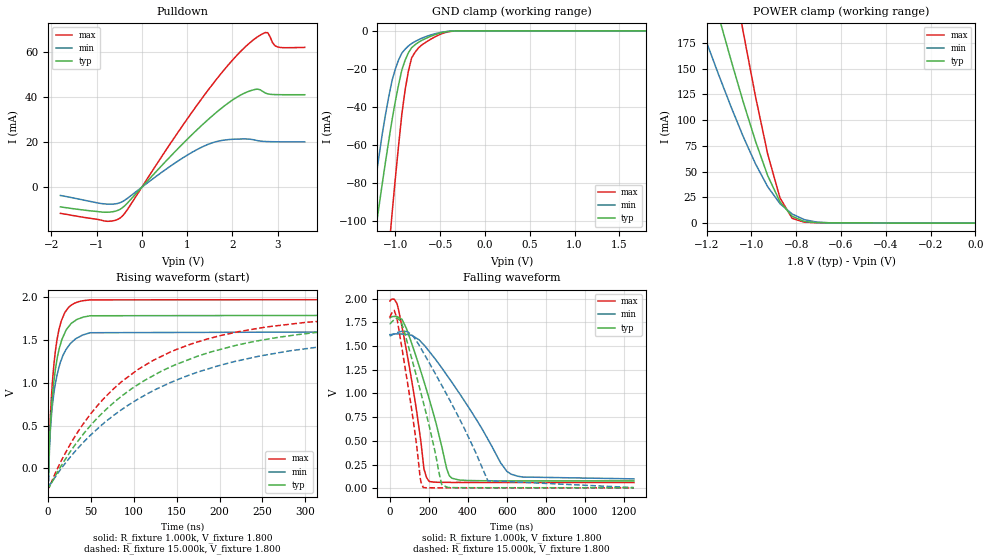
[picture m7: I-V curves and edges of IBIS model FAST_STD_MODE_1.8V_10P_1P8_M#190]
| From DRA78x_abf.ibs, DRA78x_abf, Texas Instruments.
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| Model based on original model for BI2C1833DVFZP18_SSCEV
|   Sub model FAST_STD_MODE_1.8V_10P_1P8
[model]   FAST_STD_MODE_1.8V_10P_1P8_M#190
|[Description]  [1.8V-I/O_OPEN_DRAIN-X-FAST MODE AND STD MODE, IND, 10 PERCENT%]
|   FAST MODE AND STD MODE, ,IND,10 PERCENT%
|[Input Load]
|[Output Drive] FAST MODE AND STD MODE
|Voltage   1.8V
|Mode   I/O_OPEN_DRAIN
Model_type   I/O_open_drain
Polarity   Non-Inverting
Enable   Active-Low
Vinl =  0.54
Vinh =  1.26
Cref =  15pF
Rref =  1000
Vref =  1.8V
Vmeas =  0.9
C_comp   2.29p   1.81p   2.77p
[Model Spec]
Vinl   0.54   0.486   0.594
Vinh   1.26   1.134   1.386
[Temperature Range]   25   125   -40
[Voltage Range]   1.8   1.62   1.98
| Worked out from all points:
|   slope of the pulldown table from 0 to 0.27 V, typ, clamps not added: 45.4 ohm
|   GND clamp passes 1 mA (typ) near -0.49 V on its own axis
|   POWER clamp passes 1 mA (typ) near -0.74 V on its own axis
|   rising waveform, R_fixture 1.000k, V_fixture 1.800: 20-80 % time 12.4ns typ, 14.8ns min, 10.2ns max; typ from 0.077 V to 1.8 V
|   rising waveform, R_fixture 15.000k, V_fixture 1.800: 20-80 % time 164ns typ, 193ns min, 135ns max; typ from 0.005 V to 1.73 V
|   falling waveform, R_fixture 1.000k, V_fixture 1.800: 20-80 % time 144ns typ, 283ns min, 88.9ns max; typ from 1.8 V to 0.077 V
|   falling waveform, R_fixture 15.000k, V_fixture 1.800: 20-80 % time 125ns typ, 239ns min, 77.8ns max; typ from 1.73 V to 0.005 V
[POWER_clamp]
-1.8V     746.5mA    555.3mA    1.181A
-1.218V   258.3mA    186.3mA    411.3mA
-1.127V   186.2mA    133.2mA    296.1mA
-1.055V   130.9mA    93.44mA    207.1mA
-1.036V   117.4mA    83.77mA    185.1mA
-981.8mV  79.41mA    57.45mA    122.8mA
-927.3mV  45.94mA    35.22mA    66.84mA
-872.7mV  20.67mA    18.89mA    24.46mA
-818.2mV  6.579mA    8.765mA    4.591mA
-763.6mV  1.447mA    3.292mA    765.1uA
-654.5mV  205.7uA    269.1uA    284.5uA
0V        2.27uA     701.3nA    6.122uA
[Pulldown]
-1.8V     -8.76mA    -3.66mA    -11.64mA
-763.6mV  -11.13mA   -7.517mA   -15.17mA
-490.9mV  -9.952mA   -6.962mA   -13.87mA
1.255V    26.22mA    17.12mA    37.49mA
1.691V    34.03mA    20.51mA    49.08mA
2.291V    42.09mA    21.48mA    62.55mA
2.564V    43.64mA    20.71mA    67.02mA
2.727V    41.93mA    20.35mA    68.83mA
2.782V    41.54mA    20.3mA     68.79mA
2.891V    41.26mA    20.25mA    64.24mA
3V        41.2mA     20.22mA    62.42mA
3.6V      41.16mA    20.17mA    62.23mA
[GND_clamp]
-1.8V     -312.7mA   -306.1mA   -547.2mA
-1.291V   -129.4mA   -103.7mA   -240.2mA
-1.218V   -104.5mA   -78.02mA   -197.8mA
-1.182V   -92.38mA   -65.92mA   -176.8mA
-1.073V   -57.71mA   -34.59mA   -115.9mA
-1.036V   -46.88mA   -26.15mA   -96.3mA
-927.3mV  -20.64mA   -11.73mA   -43.97mA
-890.9mV  -15.5mA    -9.682mA   -31.24mA
-818.2mV  -8.896mA   -6.689mA   -14.3mA
-672.7mV  -4.275mA   -3.291mA   -6.44mA
-381.8mV  -173.6uA   -151uA     -298.3uA
1.8V      2.27uA     911.4nA    5.692uA
[Ramp]
dV/dt_f   0.559368/0.17762757u   0.406134/0.41534074u   0.719898/0.10455527u
dV/dt_r   76.3794m/79.261671p 55.808172m/0.11582494n 92.758032m/57.986588p
R_load = 50
[Rising Waveform]
R_fixture = 1.000k
V_fixture = 1.800
V_fixture_min = 1.620
V_fixture_max = 1.980
0s        76.67mV    97.9mV     60.38mV
126ps     76.67mV    97.9mV     -142.9mV
334.9ps   -99.36mV   97.9mV     -35.5mV
768ps     77.25mV    -41.8mV    132.6mV
2.082ns   408.4mV    351.8mV    499.5mV
5.121ns   857.1mV    751mV      1.027V
12.66ns   1.385V     1.183V     1.623V
23.81ns   1.652V     1.428V     1.878V
40.96ns   1.764V     1.558V     1.956V
1.25us    1.798V     1.619V     1.974V
[Rising Waveform]
R_fixture = 15.000k
V_fixture = 1.800
V_fixture_min = 1.620
V_fixture_max = 1.980
350fs     5.398mV    6.72mV     4.165mV
147.2ps   5.398mV    6.72mV     -221.7mV
367.2ps   -210mV     6.72mV     -222.6mV
1.142ns   -213.1mV   -193.1mV   -222.1mV
45.92ns   460.5mV    353.5mV    588.3mV
104.9ns   979mV      809.5mV    1.155V
171.8ns   1.3V       1.114V     1.467V
254.1ns   1.505V     1.323V     1.649V
538.4ns   1.704V     1.558V     1.795V
1.25us    1.734V     1.608V     1.809V
[Falling Waveform]
R_fixture = 1.000k
V_fixture = 1.800
V_fixture_min = 1.620
V_fixture_max = 1.980
1.698ns   1.798V     1.619V     1.974V
23.78ns   1.812V     1.626V     1.994V
45.46ns   1.802V     1.627V     1.885V
84.51ns   1.692V     1.623V     1.47V
127.7ns   1.438V     1.595V     951.4mV
175.6ns   1.127V     1.511V     203.6mV
202.8ns   940.4mV    1.443V     71.84mV
305.5ns   131.6mV    1.156V     62.01mV
621.3ns   78.01mV    148.5mV    61.06mV
1.25us    77.48mV    98.9mV     60.85mV
[Falling Waveform]
R_fixture = 15.000k
V_fixture = 1.800
V_fixture_min = 1.620
V_fixture_max = 1.980
22.38ps   1.734V     1.609V     1.809V
23.9ns    1.778V     1.629V     1.875V
37.58ns   1.796V     1.639V     1.792V
71.85ns   1.677V     1.654V     1.365V
121.6ns   1.303V     1.601V     705.9mV
155.5ns   1.041V     1.492V     122.6mV
172.1ns   909.6mV    1.433V     7.453mV
265.8ns   43.75mV    1.088V     4.389mV
502.3ns   5.552mV    80.16mV    4.18mV
1.25us    5.398mV    6.959mV    4.165mV
